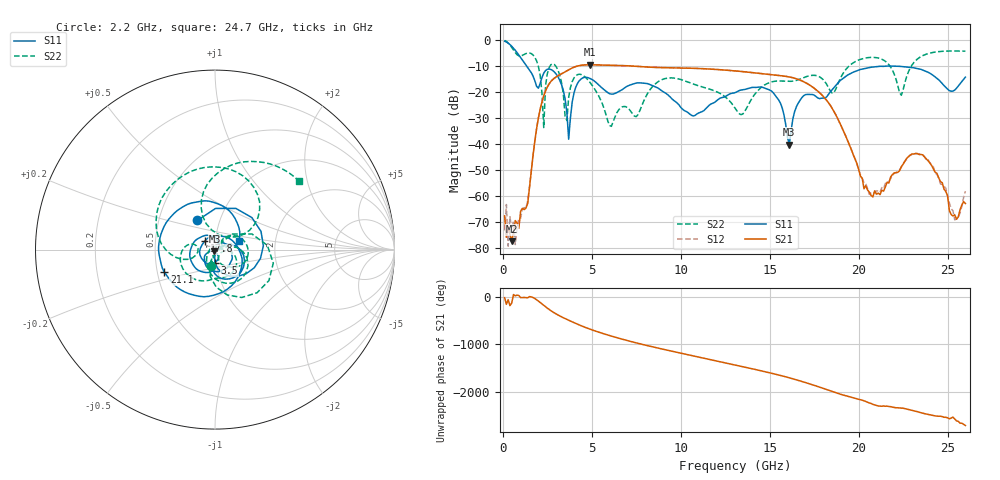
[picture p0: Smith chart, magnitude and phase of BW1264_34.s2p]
!Keysight Technologies,N5245B,MY57181159,A.13.60.06
!Date: Friday, December 18, 2020 23:53:45
!Correction: S11(Full 2 Port(1,2))
!S21(Full 2 Port(1,2))
!S12(Full 2 Port(1,2))
!S22(Full 2 Port(1,2))
!S2P File: Measurements: S11, S21, S12, S22:
# Hz S  dB  R 50
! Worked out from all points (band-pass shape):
!   260 points, 100 MHz to 26 GHz, reference 50 ohm
!   highest |S21| = -9.57 dB at 4.9 GHz (marker M1); lowest = -77.5 dB at 500 MHz (marker M2)
!   |S21| within 3 dB of the highest: 3.422 GHz to 14.02 GHz (10.59 GHz wide, 122 % of centre)
!   lowest |S11| = -40.3 dB at 16.1 GHz (marker M3), VSWR 1.02, Z = 49.7 - j0.924 ohm
!   |S11| at or under -10 dB: 1.328 GHz to end of sweep
!   |S22| runs from -33.7 to -0.2 dB; largest |S21 - S12| = 0.00078
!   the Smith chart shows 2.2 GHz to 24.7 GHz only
!   S11 on the Smith chart (normalised r, x): 2.2 GHz: 0.78, +0.26; 3.5 GHz: 0.99, -0.15; 17.8 GHz: 0.89, +0.08; 21.1 GHz: 0.55, -0.15; 24.7 GHz: 1.31, +0.13
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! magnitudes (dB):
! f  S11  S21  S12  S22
! 100 MHz  -0.5  -67.7  -73.3  -0.2
! 500 MHz  -2.4  -77.5  -73.1  -2.9
! 1.4 GHz  -10.7  -62.9  -61.9  -5.0
! 2.2 GHz  -14.5  -23.8  -23.8  -20.4
! 2.3 GHz  -12.8  -21.5  -21.5  -33.7
! 2.9 GHz  -12.3  -14.7  -14.7  -9.5
! 3.5 GHz  -22.7  -12.3  -12.3  -29.4
! 3.7 GHz  -38.2  -11.5  -11.5  -22.2
! 4.5 GHz  -14.6  -9.7  -9.7  -13.6
! 4.9 GHz  -14.8  -9.6  -9.6  -16.3
! 6.1 GHz  -20.8  -9.7  -9.7  -33.3
! 8.8 GHz  -18.9  -10.6  -10.6  -15.8
! 13.1 GHz  -20.2  -11.9  -11.9  -26.7
! 15.2 GHz  -20.3  -13.5  -13.5  -16.0
! 16.1 GHz  -40.3  -14.2  -14.2  -15.9
! 17.4 GHz  -21.0  -18.1  -18.1  -13.6
! 17.8 GHz  -22.6  -20.3  -20.3  -14.2
! 21.1 GHz  -10.2  -59.0  -58.1  -7.0
! 21.7 GHz  -10.0  -55.1  -54.5  -9.5
! 22.4 GHz  -10.2  -48.7  -49.0  -21.3
! 24.7 GHz  -16.8  -55.0  -55.7  -4.4
! 26 GHz  -14.3  -63.0  -58.2  -4.3
